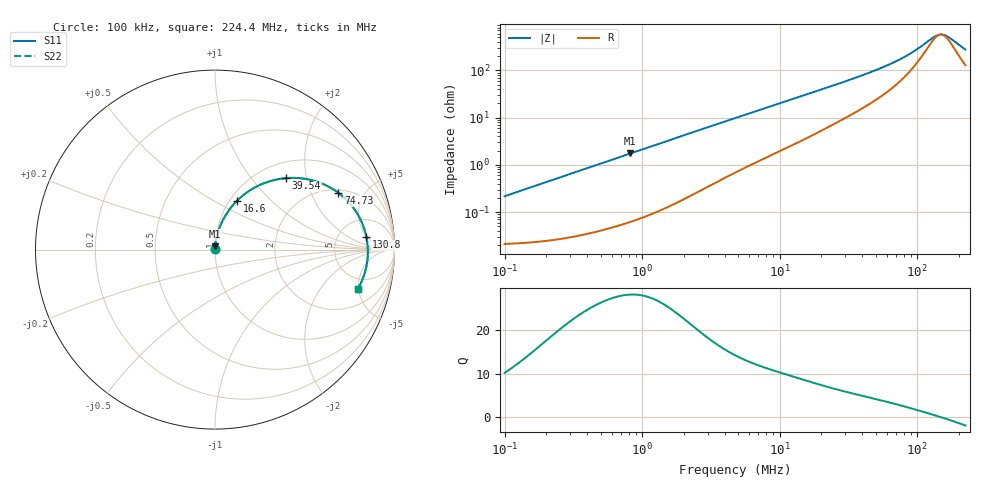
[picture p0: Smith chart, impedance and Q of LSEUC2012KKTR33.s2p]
! LSEUC2012KKTR33  S-PARAMETER MODEL  ( General Type )
! Model Generated by TAIYO YUDEN Corporation (http://www.ty-top.com)
! Version 1.0
! TAIYO YUDEN Control No. 211126
! Copyright(c) 2021 TAIYO YUDEN CO.,LTD. All Rights Reserved.
! Product Description (link to TY-COMPAS)
! https://ds.yuden.co.jp/TYCOMPAS/or/detail?pn=LSEUC2012KKTR33M&u=M
! Products Name : Inductors
! Characteristics :
!  Inductance : 0.33 uH , SRF(min) : -Hz , DC Resistance(max) : 0.024 Ohm
!  Rated Current : Saturation :5800 mA , Temp Rise : 4600 mA (40 degC)
!  Case Size : 2.0 x 1.2 / 0.079 x 0.047 [mm/inch] , Thickness : 1 / 0.039 [mm/inch]
!  (Conditions: Temperature = 25 degC , DC Bias Current/Voltage = 0A / 0V)
! External Node Assignments :
!  1  o---GGG---o  2
! GND o---------o GND
! Frequency Range : 0.1MHz  -  224.402193MHz  [ 402 STEP ]
# MHz S RI R 50
! Freq[MHz].  S11 Real  S11 Imag  S21 Real  S21 Imag  S12 Real  S12 Imag  S22 Real  S22 Imag
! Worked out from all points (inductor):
!   401 points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, 100 kHz to 224.4 MHz, reference 50 ohm
!   read as one part in series: L = 344 nH near 103.9 kHz
!   highest Q = 28.2 at 818.8 kHz (marker M1), where L = 338 nH
!   self-resonance near 148.7 MHz
!   S11 on the Smith chart (normalised r, x): 100 kHz: 1.00, +0.00; 16.6 MHz: 1.08, +0.65; 39.54 MHz: 1.31, +1.52; 74.73 MHz: 2.16, +3.20; 130.8 MHz: 10, +5; 224.4 MHz: 3.56, -4.89
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0.1  0.000217 0.00216  0.9998 -0.00216  0.9998 -0.00216  0.000217 0.00216
0.364164  0.000388 0.00781  0.9996 -0.00781  0.9996 -0.00781  0.000388 0.00781
0.818757  0.00092 0.0174  0.9991 -0.0174  0.9991 -0.0174  0.00092 0.0174
1.326154  0.00184 0.028  0.9982 -0.028  0.9982 -0.028  0.00184 0.028
2.655746  0.00589 0.0551  0.9941 -0.0551  0.9941 -0.0551  0.00589 0.0551
4.737111  0.016 0.0951  0.984 -0.0951  0.984 -0.0951  0.016 0.0951
9.671271  0.052 0.1792  0.948 -0.1792  0.948 -0.1792  0.052 0.1792
16.59799  0.1231 0.2729  0.8769 -0.2729  0.8769 -0.2729  0.1231 0.2729
17.25085  0.1306 0.2802  0.8694 -0.2802  0.8694 -0.2802  0.1306 0.2802
25.86661  0.2352 0.3531  0.7648 -0.3531  0.7648 -0.3531  0.2352 0.3531
39.54085  0.3969 0.3984  0.6031 -0.3984  0.6031 -0.3984  0.3969 0.3984
49.83986  0.5024 0.3943  0.4976 -0.3943  0.4976 -0.3943  0.5024 0.3943
62.8214  0.6109 0.3616  0.3891 -0.3616  0.3891 -0.3616  0.6109 0.3616
74.73185  0.6874 0.3164  0.3126 -0.3164  0.3126 -0.3164  0.6874 0.3164
96.03159  0.7791 0.2216  0.2209 -0.2216  0.2209 -0.2216  0.7791 0.2216
130.7541  0.8438 0.0695  0.1562 -0.0695  0.1562 -0.0695  0.8438 0.0695
143.9935  0.8509 0.0174  0.1491 -0.0174  0.1491 -0.0174  0.8509 0.0174
149.6574  0.8518 -0.0037  0.1482 0.0037  0.1482 0.0037  0.8518 -0.0037
158.5736  0.8511 -0.0354  0.1489 0.0354  0.1489 0.0354  0.8511 -0.0354
171.2936  0.8464 -0.0777  0.1536 0.0777  0.1536 0.0777  0.8464 -0.0777
211.7846  0.8111 -0.1899  0.1889 0.1899  0.1889 0.1899  0.8111 -0.1899
224.4022  0.796 -0.2186  0.204 0.2186  0.204 0.2186  0.796 -0.2186
